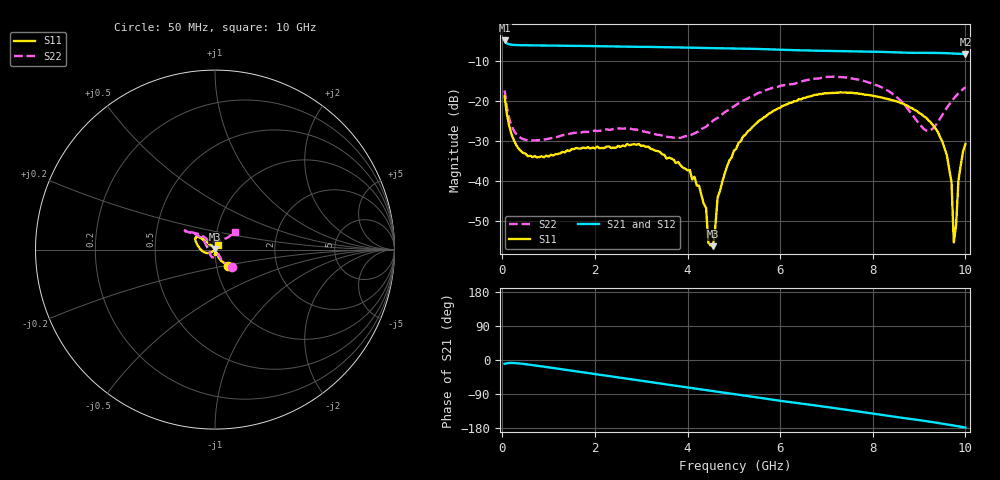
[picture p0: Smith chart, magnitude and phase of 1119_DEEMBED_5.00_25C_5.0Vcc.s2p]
!Hittite Microwave Corp.
!Digital Attenuator/PhaseShifter Rev 1.4.0
!Filename: C:\DATA\DATA\1119_DEEMBED_5.00_25C_5.0Vcc.s2p
!VNA ID: Agilent Technologies,N5224A,MY51441122,A.10.45.03
!Device type:
!2 Port Calibration.
!Temp(C): 25
!Lot Number:
!Serial Number:
!Operator:
!Misc:
!Attenuator:  5.000
# GHZ S DB R 50.0
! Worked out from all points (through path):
!   200 points, 50 MHz to 10 GHz, reference 50 ohm
!   highest |S21| = -4.97 dB at 50 MHz (marker M1); lowest = -8.4 dB at 10 GHz (marker M2)
!   group delay of S21, straight-line fit = 48.3 ps
!   lowest |S11| = -56.2 dB at 4.55 GHz (marker M3), VSWR 1.00, Z = 49.9 + j0.116 ohm
!   |S11| at or under -10 dB: start of sweep to end of sweep
!   |S22| runs from -29.9 to -14.0 dB; largest |S21 - S12| = 0.0017
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0.05  -18.87 -51.3  -4.97 -10.1  -4.97 -10.1  -17.42 -46.5
0.2  -28.38 -65.6  -6.03 -7.7  -6.04 -7.7  -26.22 -56.7
0.55  -33.78 -62.1  -6.18 -11.8  -6.18 -11.8  -29.82 -52.1
1.75  -31.61 -90.0  -6.34 -32.7  -6.34 -32.7  -27.75 -80.2
3.4  -32.68 -85.6  -6.61 -61.8  -6.62 -61.8  -28.50 -137.2
4.15  -38.88 -62.9  -6.78 -75.1  -6.80 -75.2  -28.11 175.9
4.4  -46.63 -67.7  -6.84 -79.4  -6.85 -79.5  -26.45 160.2
4.45  -55.30 -42.9  -6.86 -80.3  -6.88 -80.4  -25.91 157.7
4.55  -56.17 131.6  -6.87 -82.0  -6.90 -82.1  -24.91 152.9
4.65  -44.07 122.5  -6.89 -83.7  -6.92 -83.8  -24.24 148.6
5.05  -31.97 130.1  -6.97 -90.7  -6.99 -90.8  -20.99 140.2
5.75  -23.23 138.3  -7.17 -103.2  -7.19 -103.3  -17.09 141.7
6.7  -18.70 142.5  -7.48 -119.0  -7.50 -119.1  -14.56 147.1
7.5  -17.95 150.8  -7.66 -132.6  -7.67 -132.7  -14.33 147.2
8.35  -19.61 163.1  -7.87 -147.6  -7.87 -147.6  -17.64 137.4
9.15  -24.17 -165.6  -8.05 -161.3  -8.07 -161.3  -27.39 105.7
9.5  -30.08 -149.0  -8.10 -168.0  -8.12 -168.0  -23.52 53.6
9.7  -40.22 -137.5  -8.19 -172.0  -8.20 -172.1  -20.16 43.6
9.75  -55.24 -155.2  -8.22 -173.1  -8.23 -173.1  -19.42 42.8
9.799999  -50.83 55.8  -8.24 -174.1  -8.25 -174.1  -18.74 42.3
9.85  -39.78 59.4  -8.27 -175.1  -8.28 -175.1  -18.12 41.9
10  -30.69 57.7  -8.37 -178.2  -8.37 -178.2  -16.65 41.1
